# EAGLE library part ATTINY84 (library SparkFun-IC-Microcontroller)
Atmel 14-pin 2/4/8kB flash uC Datasheet SparkFun Products Tiny AVR Programmer (PGM-11801) SparkFun Servo Trigger - Continuous Rotation (WIG-13872) SparkFun Servo Trigger (WIG-13118)
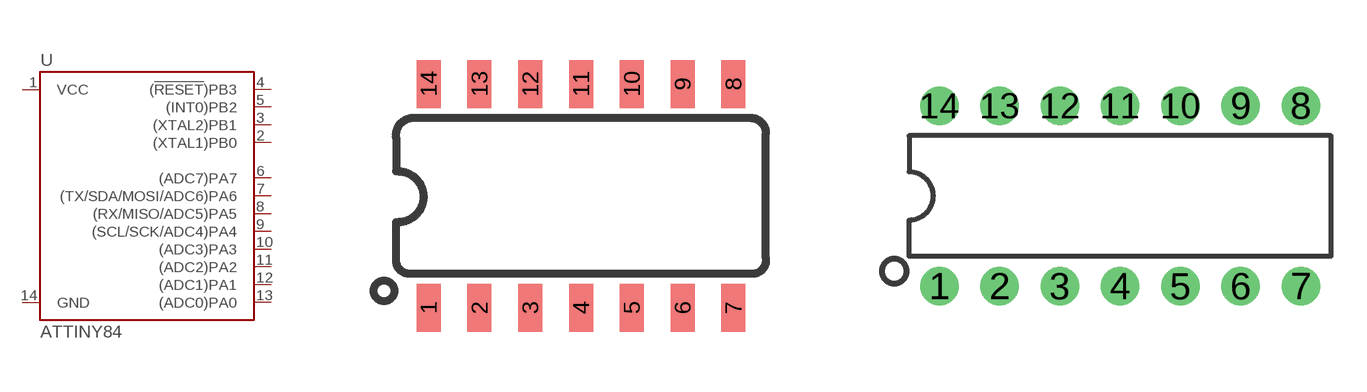
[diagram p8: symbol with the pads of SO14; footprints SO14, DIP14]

Designator prefix U

## ATTINY84 (PROD_ID: IC-11285; VALUE: ATTINY84)  [SO14]
1  VCC
2  (XTAL1)PB0
3  (XTAL2)PB1
4  (!RESET!)PB3
5  (INT0)PB2
6  (ADC7)PA7
7  (TX/SDA/MOSI/ADC6)PA6
8  (RX/MISO/ADC5)PA5
9  (SCL/SCK/ADC4)PA4
10  (ADC3)PA3
11  (ADC2)PA2
12  (ADC1)PA1
13  (ADC0)PA0
14  GND

## ATTINY84ATTINY84-20PU  [DIP14]
Pads as for SO14

## ATTINY84ATTINY84-20MU  [QFN20]
1  (SCL/SCK/ADC4)PA4
2  (ADC3)PA3
3  (ADC2)PA2
4  (ADC1)PA1
5  (ADC0)PA0
8  GND
9  VCC
11  (XTAL1)PB0
12  (XTAL2)PB1
13  (!RESET!)PB3
14  (INT0)PB2
15  (ADC7)PA7
16  (TX/SDA/MOSI/ADC6)PA6
20  (RX/MISO/ADC5)PA5

## Footprint SO14 (pad centres in mm)
SOIC, 0.15 inch width
smd 0.6 x 1.2: 1 -3.175,-2.8; 2 -1.905,-2.8; 3 -0.635,-2.8; 4 0.635,-2.8; 5 1.905,-2.8; 6 3.175,-2.8; 7 4.445,-2.8; 8 4.445,2.8; 9 3.175,2.8; 10 1.905,2.8; 11 0.635,2.8; 12 -0.635,2.8; 13 -1.905,2.8; 14 -3.175,2.8

## Footprint DIP14 (pad centres in mm)
drill 0.813 pad 1.626: 1 -7.62,-3.81; 2 -5.08,-3.81; 3 -2.54,-3.81; 4 0,-3.81; 5 2.54,-3.81; 6 5.08,-3.81; 7 7.62,-3.81; 8 7.62,3.81; 9 5.08,3.81; 10 2.54,3.81; 11 0,3.81; 12 -2.54,3.81; 13 -5.08,3.81; 14 -7.62,3.81

## Footprint QFN20 (pad centres in mm)
smd 1 x 1: 0 0,0
smd 0.65 x 0.3: 1 -1.9,1; 2 -1.9,0.5; 3 -1.9,0; 4 -1.9,-0.5; 5 -1.9,-1; 11 1.9,-1; 12 1.9,-0.5; 13 1.9,0; 14 1.9,0.5; 15 1.9,1
smd 0.3 x 0.65: 6 -1,-1.9; 7 -0.5,-1.9; 8 0,-1.9; 9 0.5,-1.9; 10 1,-1.9; 16 1,1.9; 17 0.5,1.9; 18 0,1.9; 19 -0.5,1.9; 20 -1,1.9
